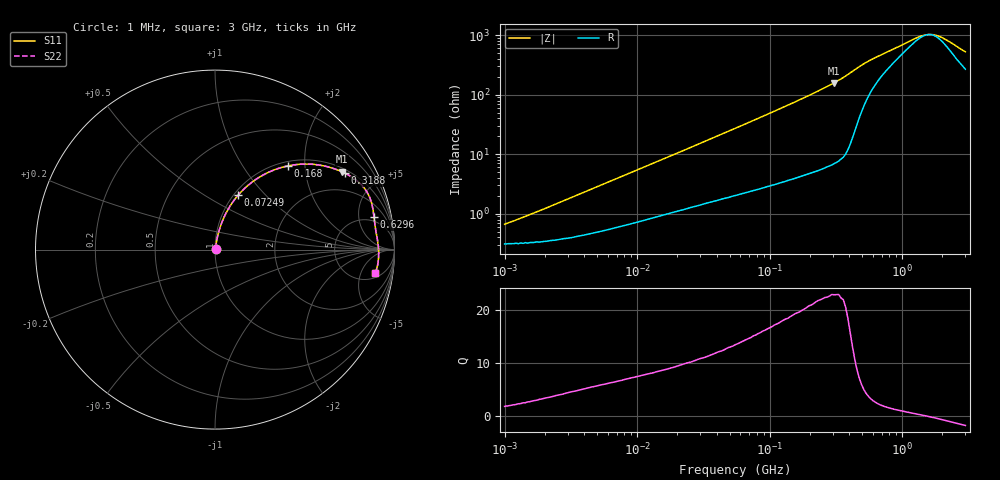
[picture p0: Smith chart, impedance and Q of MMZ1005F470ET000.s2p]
! S-parameter Generated by TDK Corporation
! Copyright(C) 2016 TDK Corporation.
! All Rights Reserved.
! TDK P/N: MMZ1005F470ET000 (Chip Beads)
! Property: |Z|=47¶ at 100MHz
! Size(LxWxT): 1x0.5x0.5mm, 0.039x0.02x0.02inches
! Model Type: s2p (Touchstone File Format Version 1.0)
! Frequency: DC=Yes Start=1MHz Stop=3000MHz 202points Log-sweep
! Note: This model was converted from impedance.
! Model Generated on May. 16, 2016
! Hash(MD5):
! Port Assignments:
!  1 ---@@@--- 2
! Applicable Conditions:
!  Temperature = 25 degC
!  DC Bias Current = 0 A
!  Small Signal Operation
! Terms and conditions regarding TDK Simulation Models
! (1)This simulation model is being provided solely for informational purposes. Please refer to the specifications of the products in terms of detailed characteristics of such products.
! (2)In no event shall TDK Corporation of any of its subsidiaries be liable for any loss or damage arising, directly or indirectly,
!  From any information contained in this simulation model, including, but not limited to loss or damages arising from any inaccuracies, omissions or errors in connection with such information.
! (3)Any and all copyrights on this simulation model are owned by TDK Corporation.
!  Duplication or redistribution of this simulation model without prior written permission from TDK Corporation is prohibited.
! (4)This simulation model is subject to any modification or change without any prior notice.
! (5)Neither TDK Corporation nor any of its subsidiaries shall make any warranty, express or implied,
!  Including but not limited to the correctness, implied warranties of merchantability and fitness for a particular purpose with respect to this simulation models.
! (6)The use of this simulation model shall be deemed to have consented to the terms and conditions hereof.
# MHz S MA R 50
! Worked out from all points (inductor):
!   201 points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, 1 MHz to 3 GHz, reference 50 ohm
!   read as one part in series: L = 92.6 nH near 1.751 MHz
!   highest Q = 22.8 at 306.3 MHz (marker M1), where L = 82.2 nH
!   self-resonance near 1.584 GHz
!   S11 on the Smith chart (normalised r, x): 1 MHz: 1.01, +0.01; 72.49 MHz: 1.05, +0.71; 168 MHz: 1.08, +1.64; 318.8 MHz: 1.15, +3.32; 629.6 MHz: 3.99, +7.91; 3 GHz: 6, -9
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1  0.006635 61.8  0.9969 -0.3  0.9969 -0.3  0.006635 61.8
1.822989  0.01111 72.0  0.9966 -0.6  0.9966 -0.6  0.01111 72.0
3.900413  0.02253 77.7  0.9954 -1.3  0.9954 -1.3  0.02253 77.7
14.61624  0.07666 78.9  0.9881 -4.4  0.9881 -4.4  0.07666 78.9
28.86629  0.1438 76.4  0.9763 -8.2  0.9763 -8.2  0.1438 76.4
54.77226  0.2572 70.9  0.9474 -14.9  0.9474 -14.9  0.2572 70.9
72.48696  0.3284 67.0  0.9226 -19.1  0.9226 -19.1  0.3284 67.0
108.1723  0.4554 59.6  0.8641 -27.0  0.8641 -27.0  0.4554 59.6
168.0187  0.619 48.9  0.7544 -38.2  0.7544 -38.2  0.619 48.9
213.6344  0.7091 42.2  0.6723 -45.1  0.6723 -45.1  0.7091 42.2
306.2963  0.8292 31.6  0.5238 -55.9  0.5238 -55.9  0.8292 31.6
318.8066  0.8409 30.3  0.5056 -57.1  0.5056 -57.1  0.8409 30.3
374.1707  0.883 25.3  0.4283 -61.9  0.4283 -61.9  0.883 25.3
439.1493  0.9072 20.1  0.3445 -64.6  0.3445 -64.6  0.9072 20.1
629.6259  0.9041 11.5  0.2139 -57.7  0.2139 -57.7  0.9041 11.5
800.5644  0.9019 8.1  0.1657 -49.8  0.1657 -49.8  0.9019 8.1
1347.129  0.9091 1.9  0.09629 -18.3  0.09629 -18.3  0.9091 1.9
1459.42  0.9104 1.0  0.09101 -9.7  0.09101 -9.7  0.9104 1.0
1645.649  0.9119 -0.5  0.0885 5.0  0.0885 5.0  0.9119 -0.5
1782.824  0.9122 -1.4  0.09099 14.6  0.09099 14.6  0.9122 -1.4
2010.32  0.9126 -3.0  0.1005 28.1  0.1005 28.1  0.9126 -3.0
3000  0.9013 -8.5  0.1716 50.8  0.1716 50.8  0.9013 -8.5
